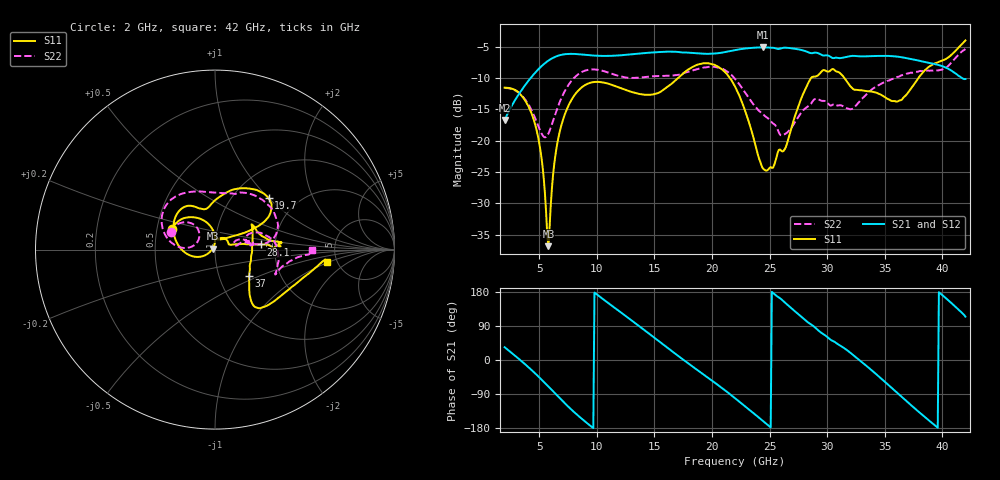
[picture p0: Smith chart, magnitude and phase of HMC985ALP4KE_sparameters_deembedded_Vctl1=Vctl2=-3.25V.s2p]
!s2p File: Measurements: S11, S21, S12, S22
# GHz S dB R 50.0
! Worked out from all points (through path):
!   401 points, 2 GHz to 42 GHz, reference 50 ohm
!   highest |S21| = -5.11 dB at 24.4 GHz (marker M1); lowest = -16.7 dB at 2 GHz (marker M2)
!   lowest |S11| = -36.8 dB at 5.8 GHz (marker M3), VSWR 1.03, Z = 48.7 + j0.578 ohm
!   |S11| at or under -10 dB: start of sweep to 17.07 GHz; 21.55 GHz to 28.61 GHz (7.054 GHz wide, 28.1 % of centre); 31.5 GHz to 37.93 GHz (6.428 GHz wide, 18.5 % of centre)
!   |S22| runs from -19.5 to -5.4 dB; largest |S21 - S12| = 0.00056
!   S11 on the Smith chart (normalised r, x): 2 GHz: 0.60, +0.15; 19.7 GHz: 1.45, +1.00; 28.1 GHz: 1.68, +0.10; 37 GHz: 1.39, -0.43; 42 GHz: 4.16, -0.99
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2  -11.54 153.8  -16.72 33.7  -16.72 33.7  -11.59 158.5
4.5  -16.49 105.0  -9.48 -31.0  -9.48 -31.0  -15.76 129.4
5.1  -21.43 92.0  -8.29 -48.5  -8.30 -48.5  -18.45 136.6
5.8  -36.84 155.6  -7.22 -70.1  -7.22 -70.1  -18.88 165.1
6.8  -18.45 -160.6  -6.36 -101.3  -6.36 -101.4  -13.77 175.5
8.7  -11.49 150.5  -6.25 -155.2  -6.25 -155.2  -9.05 146.4
10.5  -10.69 124.9  -6.48 161.6  -6.48 161.6  -8.85 120.0
12.6  -11.98 112.5  -6.30 114.0  -6.30 114.0  -9.94 92.3
15.4  -12.35 97.8  -5.86 49.6  -5.86 49.6  -9.68 71.5
17.5  -9.27 74.5  -5.94 1.1  -5.94 1.1  -9.27 67.0
19.7  -7.65 43.7  -6.14 -47.8  -6.14 -47.8  -8.23 39.5
22  -11.34 28.5  -5.55 -100.8  -5.55 -100.8  -10.13 8.9
24.4  -24.38 67.0  -5.11 -160.2  -5.11 -160.2  -15.78 14.7
26.1  -21.72 23.3  -5.20 158.2  -5.20 158.1  -19.16 17.5
28.1  -11.80 6.4  -5.71 105.2  -5.71 105.2  -14.85 16.6
28.7  -9.83 1.3  -6.04 91.9  -6.04 91.9  -13.82 14.0
30.6  -8.66 5.3  -6.82 48.6  -6.81 48.6  -14.15 11.5
32.4  -11.88 24.1  -6.48 9.4  -6.48 9.4  -14.62 22.5
35.4  -13.46 9.7  -6.49 -68.2  -6.48 -68.2  -10.38 14.1
37  -12.39 -37.6  -6.87 -111.6  -6.87 -111.6  -9.28 3.5
39.5  -7.59 -50.1  -7.84 -176.0  -7.84 -176.1  -8.78 -21.8
42  -4.01 -6.5  -10.16 114.4  -10.16 114.4  -5.37 -0.5
